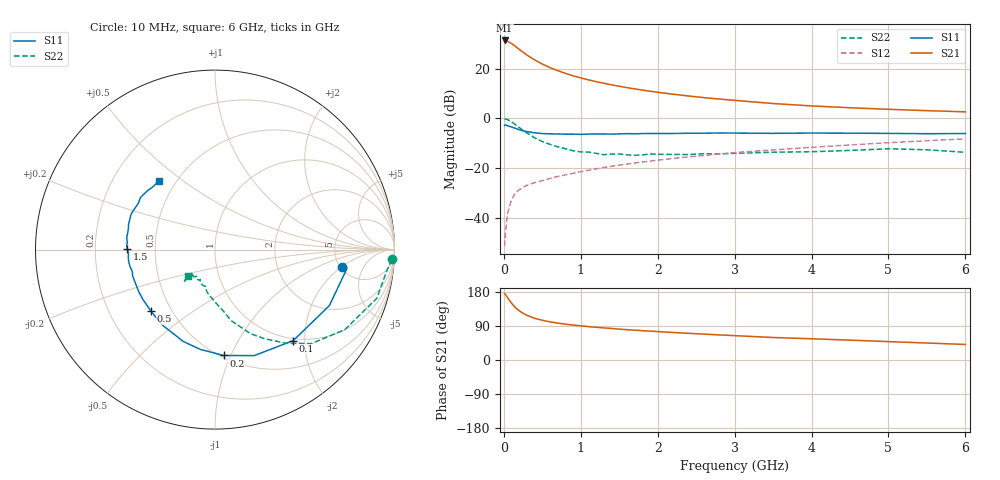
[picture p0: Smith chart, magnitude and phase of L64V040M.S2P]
!  INFINEON TECHNOLOGIES Small Signal Semiconductors
! BFR380L3 , Si-NPN RF-Transistor in TSLP-3-1
!  Vce=4 V,  Ic=40 mA
! Common Emitter S-Parameters:  07. March 2005
#  GHz  S  MA  R  50
! f  S11  S21  S12  S22
! GHz  Mag  Ang  Mag  Ang  Mag  Ang  Mag  Ang
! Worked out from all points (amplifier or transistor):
!   36 points, 10 MHz to 6 GHz, reference 50 ohm
!   highest |S21| = 31.3 dB at 10 MHz (marker M1)
!   |S21| within 3 dB of that: start of sweep to 176.4 MHz
!   unconditionally stable (mu >= 1): 1.884 GHz to 4.817 GHz
!   at 250 MHz: K = 0.41, MSG = 27.2 dB, |S12| = -27.8 dB
!   at 1.4 GHz: K = 0.96, MSG = 16.4 dB, |S12| = -19.3 dB
!   at 6 GHz: K = 0.98, MSG = 5.4 dB, |S12| = -8.2 dB
!   S11 on the Smith chart (normalised r, x): 10 MHz: 5.19, -2.03; 100 MHz: 0.96, -1.76; 200 MHz: 0.52, -0.94; 500 MHz: 0.39, -0.35; 1.5 GHz: 0.34, +0.00; 6 GHz: 0.40, +0.41
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0.01  0.7149 -7.7  36.76 174.8  0.0027 78.3  0.9862 -3.2
0.02  0.7432 -8.0  36.71 173.5  0.005 87.0  0.9656 -6.8
0.05  0.7096 -26.1  35.29 163.8  0.0125 80.1  0.9412 -16.8
0.1  0.6686 -49.3  31.83 149.9  0.0233 68.5  0.8494 -31.7
0.15  0.6299 -69.7  28.04 138.4  0.0315 61.9  0.7501 -44.3
0.2  0.5916 -85.4  24.34 129.8  0.0368 58.3  0.6551 -52.8
0.25  0.5621 -98.3  21.32 123.3  0.0408 55.3  0.5682 -60.9
0.3  0.5415 -109.0  18.7 117.9  0.0451 54.0  0.5097 -67.0
0.4  0.5126 -125.2  14.96 110.1  0.0512 53.7  0.4065 -77.1
0.5  0.4945 -136.4  12.36 104.8  0.056 54.3  0.3418 -82.7
0.6  0.4884 -145.1  10.45 100.6  0.0621 55.3  0.3 -88.6
0.8  0.4813 -157.3  8.029 94.6  0.0731 57.6  0.2453 -99.7
0.9  0.4816 -162.5  7.161 92.2  0.0786 58.8  0.2235 -103.6
1.1  0.4833 -169.1  5.936 88.1  0.0904 61.1  0.2101 -109.4
1.5  0.4883 179.7  4.414 81.4  0.1149 63.3  0.1928 -119.7
1.8  0.4942 173.4  3.702 77.4  0.1324 64.0  0.184 -125.2
2.2  0.4963 166.6  3.058 72.6  0.1563 64.4  0.1882 -128.6
2.8  0.5072 157.5  2.443 66.2  0.192 64.6  0.1924 -135.6
3.5  0.4993 148.7  1.985 59.4  0.232 62.9  0.2086 -134.8
4.5  0.503 142.5  1.633 52.4  0.2927 61.6  0.227 -134.6
5.5  0.4914 134.3  1.427 44.8  0.3551 58.1  0.2336 -134.2
6  0.4954 129.2  1.352 41.0  0.3874 56.0  0.2079 -135.8
